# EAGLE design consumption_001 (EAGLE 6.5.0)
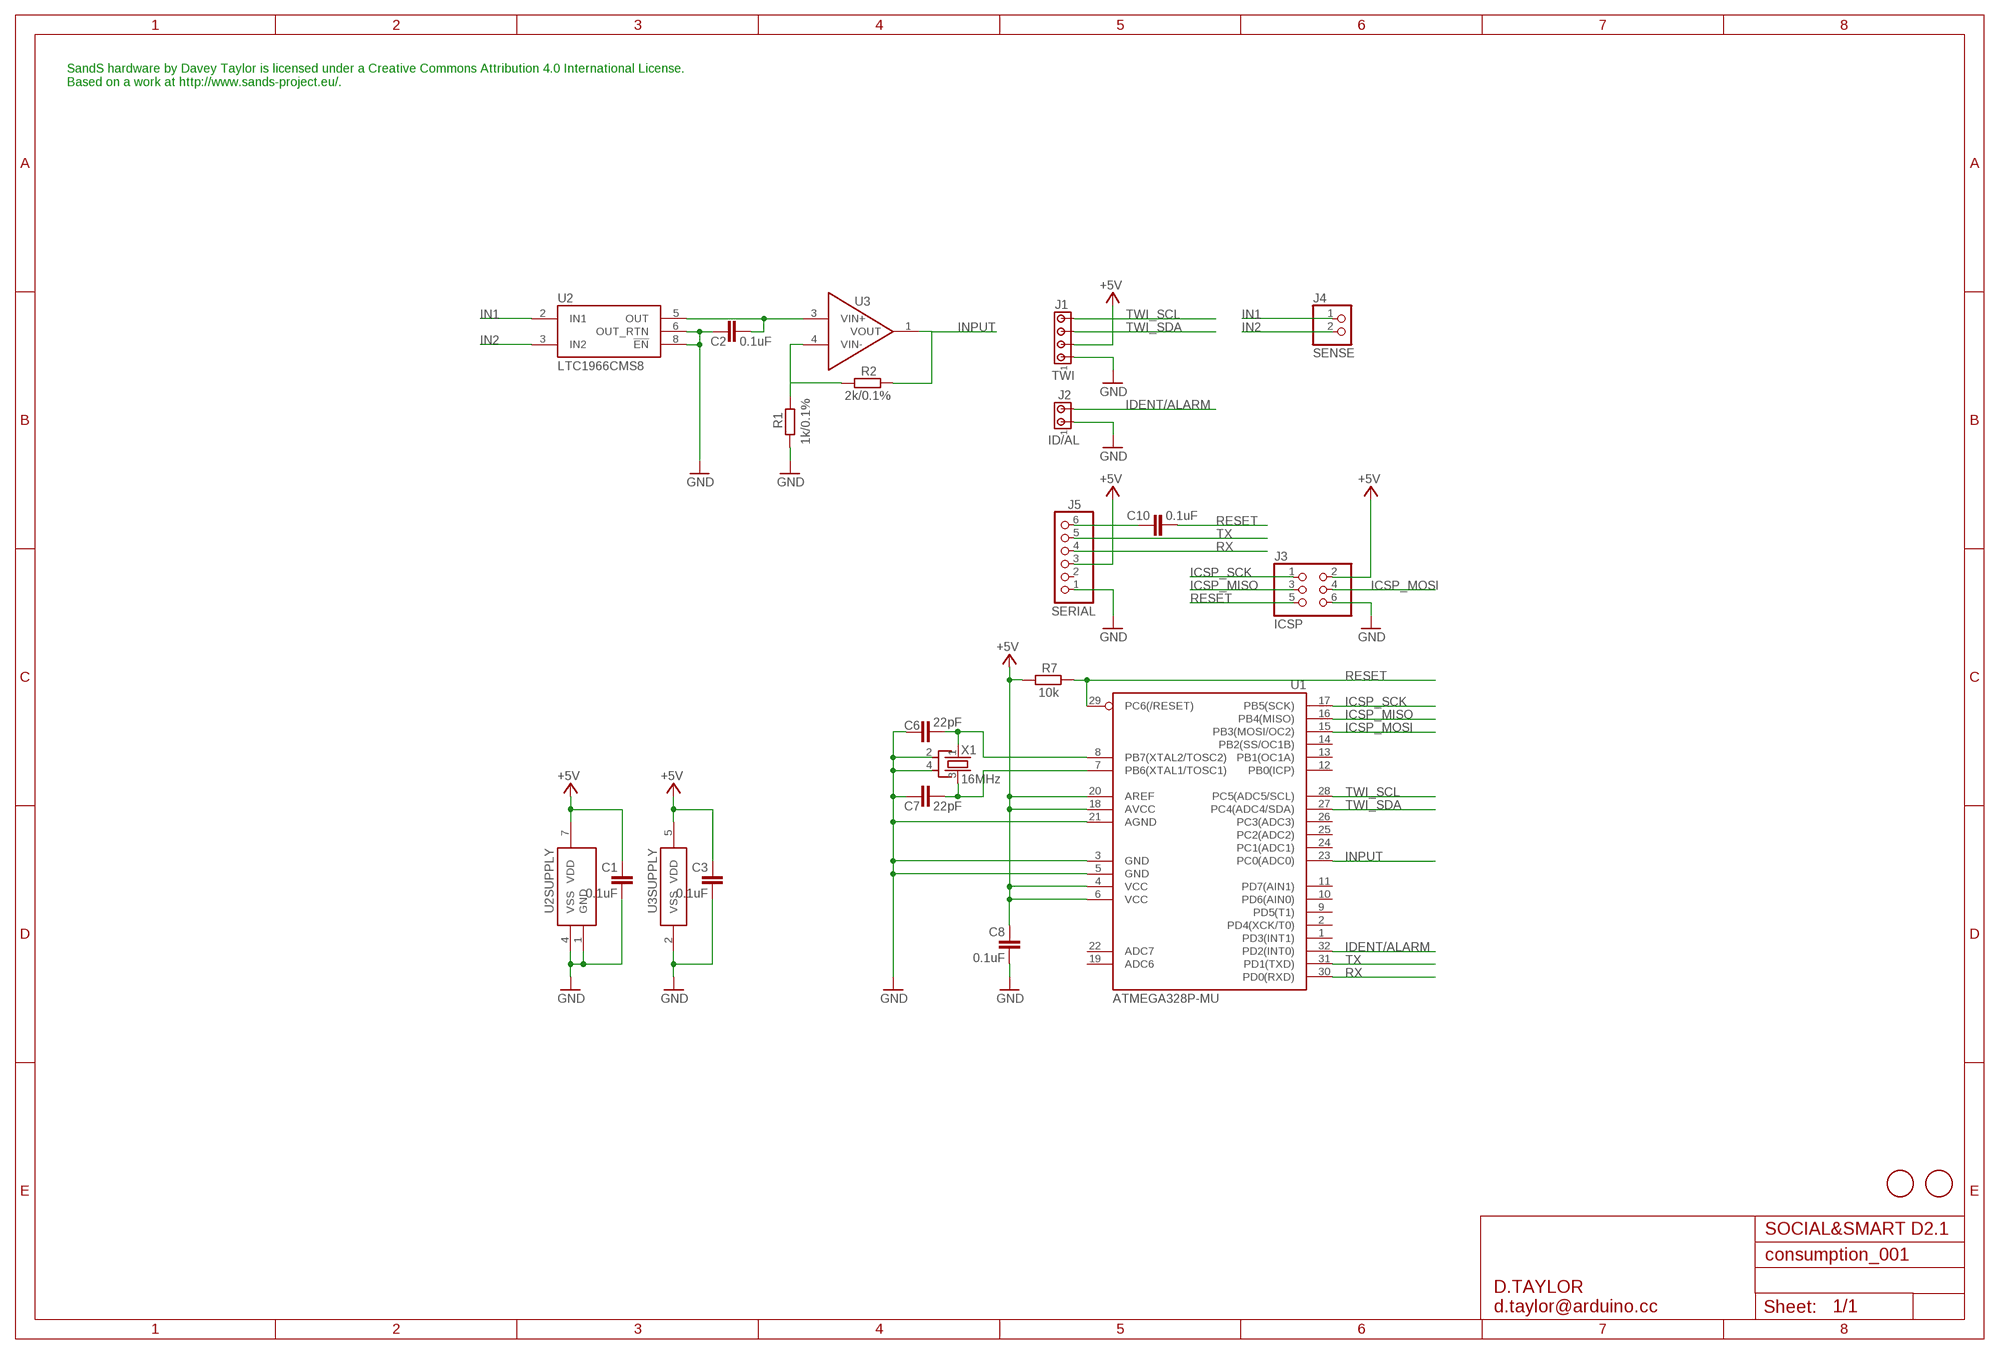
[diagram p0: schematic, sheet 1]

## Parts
C1  0.1uF  C-EUC0603  [C0603]
C2  0.1uF  C-EUC0603  [C0603]
C3  0.1uF  C-EUC0603  [C0603]
C6  22pF  C-EUC0603  [C0603]
C7  22pF  C-EUC0603  [C0603]
C8  0.1uF  C-EUC0603  [C0603]
C10  0.1uF  C-EUC0603  [C0603]
J1  TWI  MTA04-100  [10X04MTA]
J2  ID/AL  MTA02-100  [10X02MTA]
J3  ICSP  PINHD-2X3  [2X03]
J4  SENSE  MKDS_1,5/2-5,08  [MKDS1,5/2-5,08]
J5  SERIAL  PINHD-1X6  [1X06]
R1  1k/0.1%  R-EU_R0603  [R0603]
R2  2k/0.1%  R-EU_R0603  [R0603]
R7  10k  R-EU_R0603  [R0603]
U1  ATMEGA328P-MU  [MLF32-M1-A]
U2  LTC1966CMS8  [MSOP08]
U3  MCP6401-E/OT  [SOT-23-5]
U$5  FIDUCIALMOUNT  [FIDUCIA-MOUNT]
U$6  FIDUCIALMOUNT  [FIDUCIA-MOUNT]
X1  16MHz  CRYSTAL-KX7  [XTAL-3.2-2.5]

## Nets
+5V: C1.1 C3.1 C8.1 J1.2 J3.2 J5.3 R7.1 U1.4(VCC) U1.6(VCC) U1.18(AVCC) U1.20(AREF) U2.7(VDD) U3.5(VDD)
GND: C1.2 C2.1 C3.2 C6.1 C7.1 C8.2 J1.1 J2.1 J3.6 J5.1 R1.1 U1.3(GND) U1.5(GND) U1.21(AGND) U2.1(GND) U2.4(VSS) U2.6(OUT_RTN) U2.8(!EN!) U3.2(VSS) X1.2(SH1) X1.4(SH2)
ICSP_MISO: J3.3 U1.16(PB4(MISO))
ICSP_MOSI: J3.4 U1.15(PB3(MOSI/OC2))
ICSP_SCK: J3.1 U1.17(PB5(SCK))
IDENT/ALARM: J2.2 U1.32(PD2(INT0))
IN1: J4.1 U2.2(IN1)
IN2: J4.2 U2.3(IN2)
INPUT: R2.1 U1.23(PC0(ADC0)) U3.1(VOUT)
N$1: C2.2 U2.5(OUT) U3.3(VIN+)
N$2: R1.2 R2.2 U3.4(VIN-)
N$6: C6.2 U1.8(PB7(XTAL2/TOSC2)) X1.1(X1)
N$7: C7.2 U1.7(PB6(XTAL1/TOSC1)) X1.3(X2)
N$9: C10.1 J5.6
RESET: C10.2 J3.5 R7.2 U1.29(PC6(/RESET))
RX: J5.4 U1.30(PD0(RXD))
TWI_SCL: J1.4 U1.28(PC5(ADC5/SCL))
TWI_SDA: J1.3 U1.27(PC4(ADC4/SDA))
TX: J5.5 U1.31(PD1(TXD))
Unconnected: J5.2 U1.1(PD3(INT1)) U1.2(PD4(XCK/T0)) U1.9(PD5(T1)) U1.10(PD6(AIN0)) U1.11(PD7(AIN1)) U1.12(PB0(ICP)) U1.13(PB1(OC1A)) U1.14(PB2(SS/OC1B)) U1.19(ADC6) U1.22(ADC7) U1.24(PC1(ADC1)) U1.25(PC2(ADC2)) U1.26(PC3(ADC3))

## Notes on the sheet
- SandS hardware by Davey Taylor is licensed under a Creative Commons Attribution 4.0 International License.
  Based on a work at http://www.sands-project.eu/.
- SOCIAL&SMART D2.1
- D.TAYLOR
  d.taylor@arduino.cc

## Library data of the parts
C1-C3 C6-C8 C10 = rcl:C-EU: CAPACITOR, European symbol
J1 = con-amp:MTA04-100: AMP connector
J2 = con-amp:MTA02-100: AMP connector
J3 = pinhead:PINHD-2X3: PIN HEADER
J4 = d_taylor:MKDS_1,5/2-5,08: Screw terminal header
J5 = pinhead:PINHD-1X6: PIN HEADER
R1 R2 R7 = rcl:R-EU_: RESISTOR, European symbol
U1 = d_taylor:ATMEGA*: MICROCONTROLLER 8 Kbytes FLASH 1 kbytes SRAM 512 bytes EEPROM USART 6-channel 10 bit ADC 2-channel 8 bit ADC Source: avr.lbr
U2 = d_taylor:LTC1966*MS8: Precision Micropower Delta-Sigma RMS-to-DC Converter
U3 = d_taylor:MCP6401*
U$5 U$6 = SmartPrj:FIDUCIALMOUNT
X1 = d_taylor:CRYSTAL-KX7

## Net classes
1 PWR: width 0.406 mm, clearance 0.254 mm

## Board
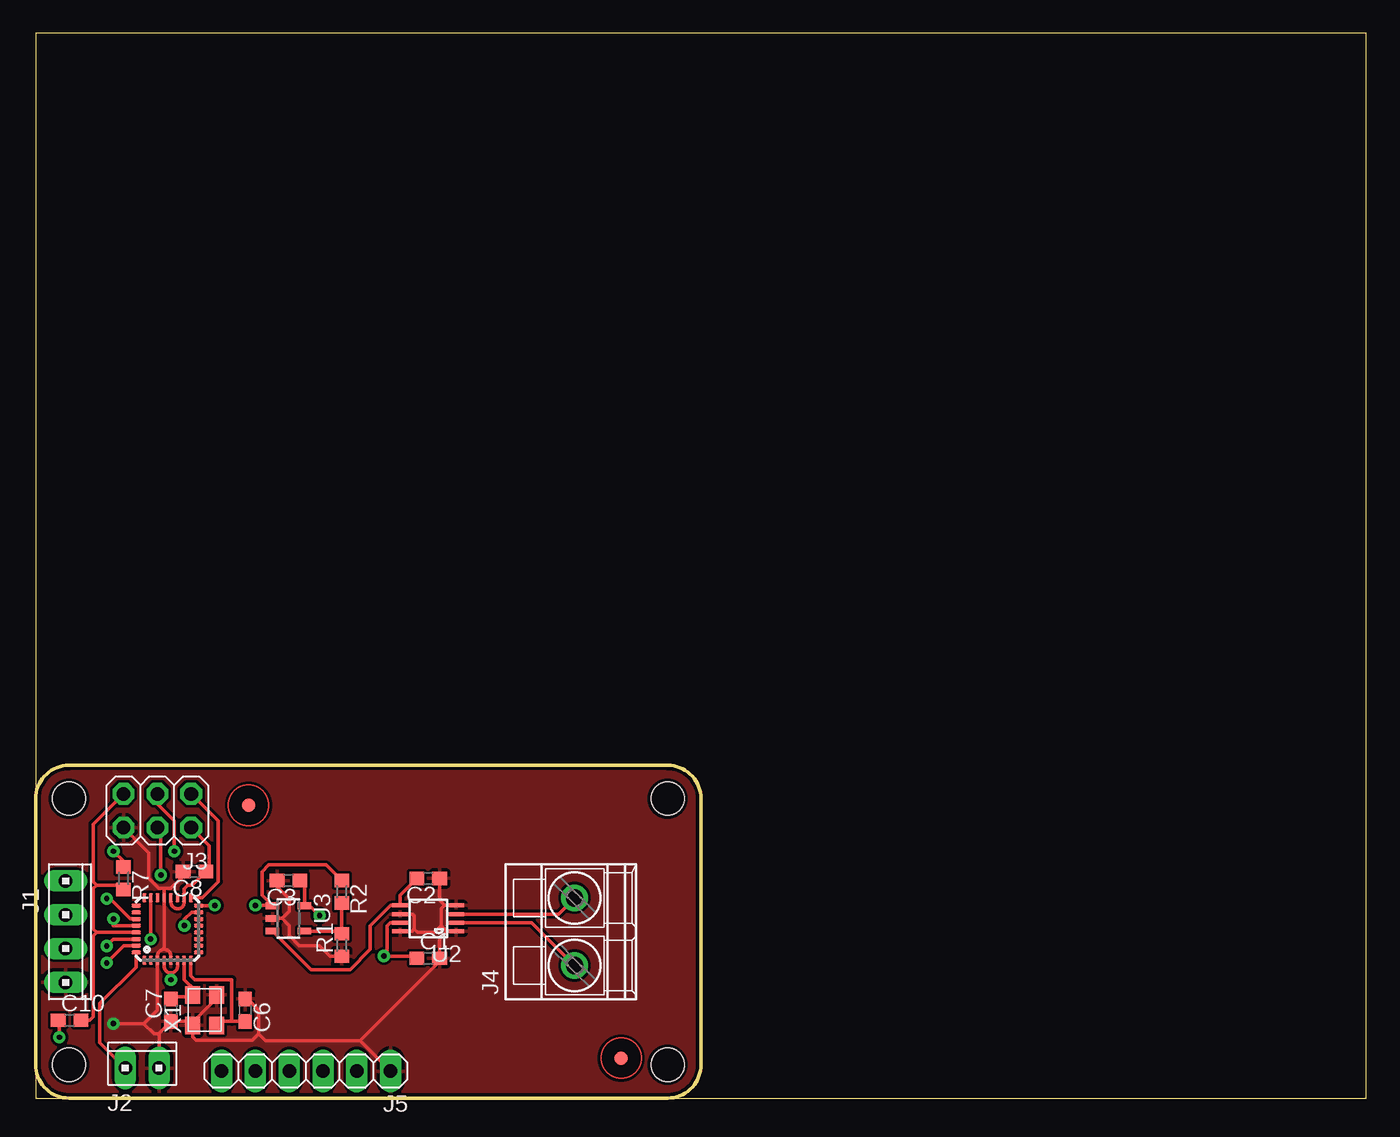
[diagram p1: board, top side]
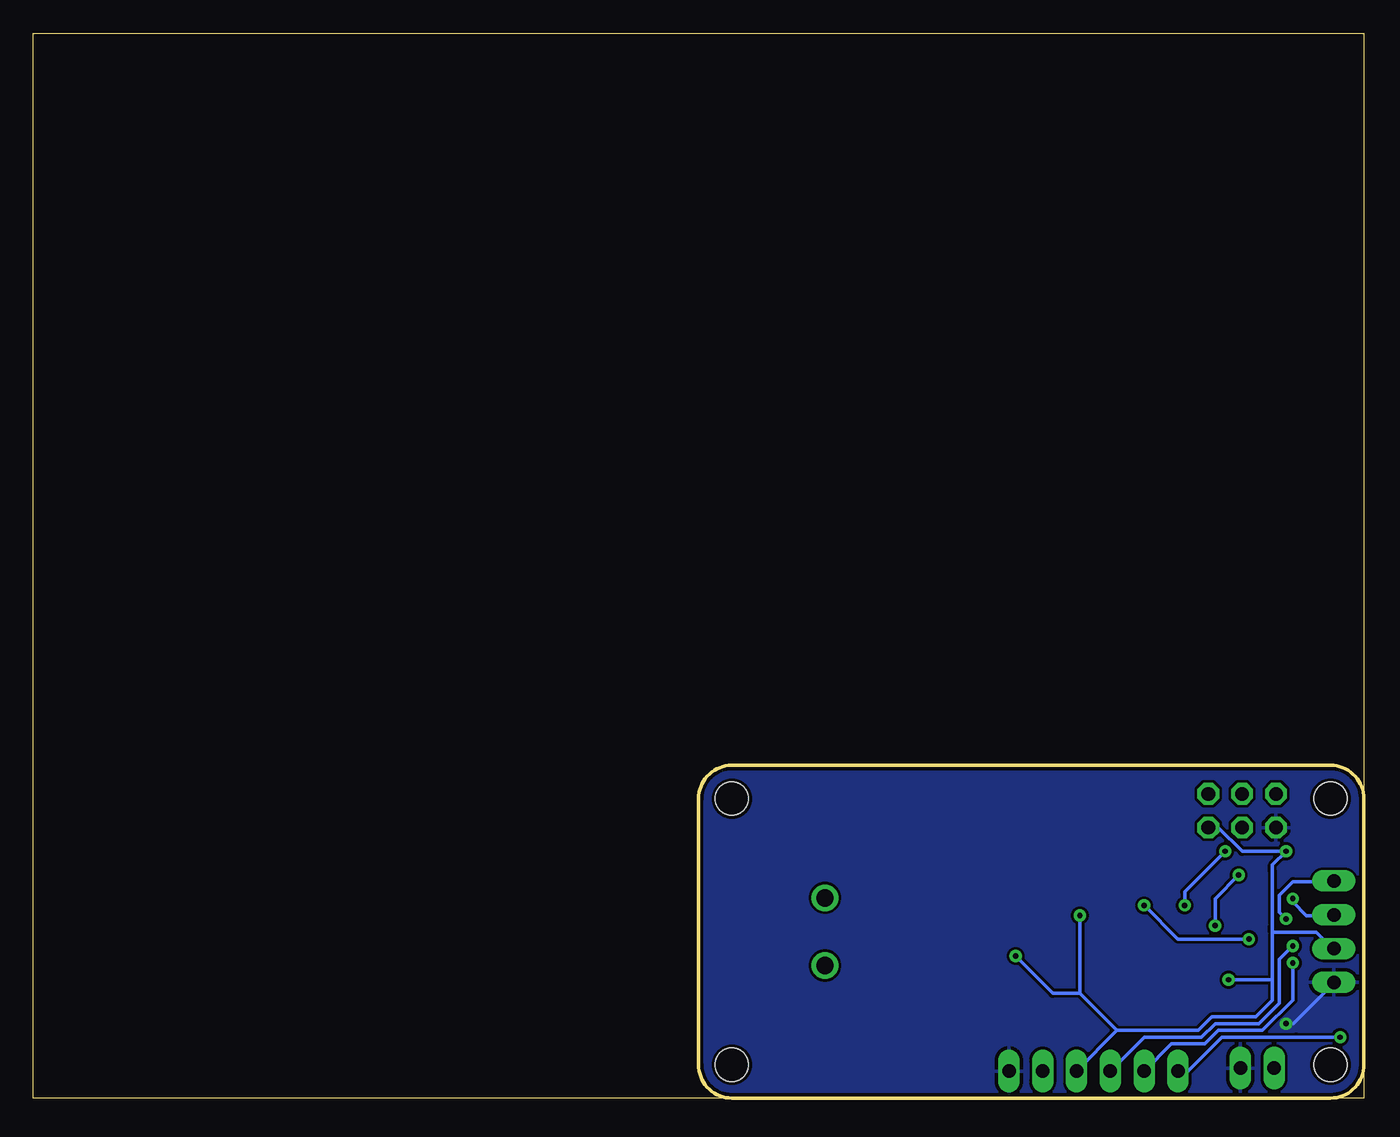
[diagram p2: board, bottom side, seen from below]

Size 100 x 80 mm. Coordinates in mm from the lower left corner, seen from the top.
Outline: 0,0 100,0 100,80 0,80 0,0
Outline: 2.5,0 47.5,0 arc90 50,2.5 50,22.5 arc90 47.5,25 2.5,25 arc90 0,22.5 0,2.5 arc90 2.5,0
Copper layers (1*16): Top 0.035mm / dielectric 1.5mm / Bottom 0.035mm
Design rules "smartprj-mini *": minimum track width 8mil, minimum drill 16mil, track to track 8mil, track to pad 8mil, pad to pad 0.200659375mm, via to via 8mil, smd to smd 4mil, copper to edge 10mil, drill to drill 8mil, minimum pad ring 12mil, minimum via ring 10mil, stop-mask expansion 2mil, vias tented up to drill 20mil, thermal gap 10mil
Holes 2.5 mm at 2.5,22.5 2.5,2.5 47.5,2.5 47.5,22.5

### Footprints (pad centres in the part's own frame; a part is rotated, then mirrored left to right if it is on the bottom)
C0603 = smd 1.1 x 1: 1 -0.85,0; 2 0.85,0
10X04MTA = drill 1.016 long: 1 3.81,0; 2 1.27,0; 3 -1.27,0; 4 -3.81,0
10X02MTA = drill 1.016 long: 1 1.27,0; 2 -1.27,0
2X03 = drill 1.016 octagon: 1 -2.54,-1.27; 2 -2.54,1.27; 3 0,-1.27; 4 0,1.27; 5 2.54,-1.27; 6 2.54,1.27
MKDS1,5/2-5,08 = drill 1.3 pad 2: 1 -2.54,0; 2 2.54,0
1X06 = drill 1.016 long: 1 -6.35,0; 2 -3.81,0; 3 -1.27,0; 4 1.27,0; 5 3.81,0; 6 6.35,0
R0603 = smd 1 x 1.1: 1 -0.85,0; 2 0.85,0
MLF32-M1-A = smd 0.7 x 0.3: 1 -2.35,1.75; 2 -2.35,1.25; 3 -2.35,0.75; 4 -2.35,0.25; 5 -2.35,-0.25; 6 -2.35,-0.75; 7 -2.35,-1.25; 8 -2.35,-1.75; 17 2.35,-1.75; 18 2.35,-1.25; 19 2.35,-0.75; 20 2.35,-0.25; 21 2.35,0.25; 22 2.35,0.75; 23 2.35,1.25; 24 2.35,1.75 | smd 0.3 x 0.7: 9 -1.75,-2.35; 10 -1.25,-2.35; 11 -0.75,-2.35; 12 -0.25,-2.35; 13 0.25,-2.35; 14 0.75,-2.35; 15 1.25,-2.35; 16 1.75,-2.35; 25 1.75,2.35; 26 1.25,2.35; 27 0.75,2.35; 28 0.25,2.35; 29 -0.25,2.35; 30 -0.75,2.35; 31 -1.25,2.35; 32 -1.75,2.35
MSOP08 = smd 0.3 x 1.2: 1 -0.976,-2.113; 2 -0.326,-2.113; 3 0.324,-2.113; 4 0.974,-2.113; 5 0.974,2.112; 6 0.324,2.112; 7 -0.326,2.112; 8 -0.976,2.112
SOT-23-5 = smd 0.5 x 1: 1 -0.95,-1.2; 2 0,-1.2; 3 0.95,-1.2; 4 0.95,1.2; 5 -0.95,1.2
FIDUCIA-MOUNT = smd 1.016 x 1.016: P$1 0,0
XTAL-3.2-2.5 = smd 1.3 x 1.1: 1 -1.15,-0.9; 2 1.15,-0.9; 3 1.15,0.9; 4 -1.15,0.9

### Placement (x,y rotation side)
C1  29.5,10.5 0 top
C2  29.5,16.5 180 top
C3  19,16.34 180 top
C6  15.75,6.6 270 top
C7  10.16,6.6 90 top
C8  11.94,17.02 180 top
C10  2.54,5.84 0 top
J1  2.25,12.5 270 top
J2  8,2.25 0 top
J3  9.14,21.59 180 top
J4  40.5,12.5 90 top
J5  20.32,2.03 180 top
R1  23,11.5 90 top
R2  23,15.5 270 top
R7  6.6,16.51 270 top
U1  9.91,12.7 90 top
U2  29.5,13.5 90 top
U3  19,13.5 270 top
U$5  16,22 0 top
U$6  44,3 0 top
X1  12.7,6.6 90 top

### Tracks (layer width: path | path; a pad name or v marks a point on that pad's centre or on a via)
+5V  (via drill 0.41)
  Top 0.254: 11.18,15.32 U1.18 | 11.18,15.05 U1.18 | R7.1 6.6,17.78 v5.84,18.54 | U1.4 9.66,9.9 arc90 10.16,9.4 | 10.16,9.4 arc90 10.66,9.89 U1.6 | 10.16,9.4 v10.16,8.89 | U1.18 11.16,15.64 11.16,15.73 11.43,16 11.77,16 C8.1 13.04,17.27 13.04,18.96 J3.2 | U1.18 11.16,14.71 arc-90 10.67,14.22 arc-90 10.16,14.74 U1.20 | C3.1 20.2,15.99 U3.5 20.6,14.45 v21.34,13.72 | U2.7 26.64,13.17 26.42,12.95 26.42,12.19 26.42,10.92 v26.16,10.67 28.48,10.67 C1.1
  Bottom 0.254: 18.54,5.08 12.45,5.08 11.43,6.1 8.13,6.1 7.37,6.86 6.86,7.37 6.86,8.89 | 6.86,15.75 6.86,15.49 | 6.86,15.49 6.86,12.95 | 6.86,12.95 6.86,12.45 | 6.86,12.45 3.56,12.45 2.25,11.18 J1.2 | 6.86,12.45 6.86,12.95 | 6.86,12.95 6.86,8.89 | 6.86,15.75 6.86,17.02 6.86,17.53 v5.84,18.54 9.14,18.54 10.92,20.32 J3.2 | J5.3 18.54,5.08 | v10.16,8.89 6.86,8.89 | 6.86,15.75 6.86,15.49 | v21.34,13.72 21.34,7.87 | 21.34,7.87 18.54,5.08 | 21.34,7.87 23.37,7.87 v26.16,10.67
GND  (via drill 0.41)
  Top 0.254: 13.85,7.62 X1.2 13.6,7.5 12.7,6.6 11.8,5.7 X1.4 | 12.05,5.75 X1.4 | 10.16,10.16 U1.5 10.16,10.68 arc90 9.66,11.18 | 9.14,10.35 U1.3 9.14,10.35 | 9.66,11.18 9.65,11.18 U1.21 9.65,15.75 | 9.14,10.35 9.14,6.6 8.13,5.59 | J2.1 9.27,4.06 9.27,4.35 9.27,4.83 | X1.4 11.8,5.75 C7.1 9.27,4.86 9.27,4.83 | 9.14,10.35 9.14,10.66 arc-90 9.66,11.18 | C6.1 15.91,7.45 16.76,6.6 16.76,4.83 | 16.76,4.83 16.26,4.35 12.05,4.35 11.8,4.6 X1.4 | J3.6 8.5,18.42 8.5,16.5 9.25,15.75 9.65,15.75 | 9.65,15.75 10.16,15.75 10.92,16.51 10.92,16.85 C8.2 | 8.13,5.59 v5.84,5.59 | 8.13,5.59 8.89,4.83 9.27,4.83 | U2.4 30.73,14.48 | 30.73,14.48 30.48,14.22 30.48,12.95 | U2.1 30.91,12.52 | 30.91,12.52 30.48,12.95 | 30.91,12.52 30.35,11.96 C1.2 30.35,10.28 24.38,4.32 | 30.73,14.48 30.35,14.86 C2.1 | U2.6 28.34,13.82 28.45,13.72 28.45,12.7 | U2.8 28.27,12.52 28.45,12.7 | 28.45,12.7 28.7,12.45 29.97,12.45 30.48,12.95 | 16.76,4.83 17.27,4.32 24.38,4.32 | 24.38,4.32 J5.1 | R1.1 22.12,10.65 21.34,11.43 19.84,11.43 19.81,11.46 19.08,12.19 19.05,12.19 19.05,12.95 18.5,13.5 | U3.2 18.5,13.5 | C3.2 18.15,15.89 19.05,14.99 19.05,14.05 18.5,13.5
  Bottom 0.254: 2.25,8.64 5.3,5.59 v5.84,5.59
  pour Top: 0.5,22.5 arc-90 2.5,24.5 47.5,24.5 arc-90 49.5,22.5 49.5,2.5 arc-90 47.5,0.5 2.5,0.5 arc-90 0.5,2.5
  pour Bottom: 0.5,22.5 arc-90 2.5,24.5 47.5,24.5 arc-90 49.5,22.5 49.5,2.5 arc-90 47.5,0.5 2.5,0.5 arc-90 0.5,2.5
ICSP_MISO  (via drill 0.41)
  Top 0.254: J3.3 9.14,22.1 10.41,20.83 10.41,19.56 v10.41,18.54 | v13.46,14.48 13.72,14.45 U1.16
  Bottom 0.254: v10.41,18.54 13.46,15.49 v13.46,14.48
ICSP_MOSI  (via drill 0.41)
  Top 0.254: J3.4 9.4,20.07 v9.4,16.76 | U1.15 11.7,13.95 11.18,13.42 v11.18,12.95
  Bottom 0.254: v9.4,16.76 11.18,14.99 v11.18,12.95
ICSP_SCK
  Top 0.254: U1.17 12.51,15.05 13.72,16.26 13.72,20.83 J3.1
IDENT/ALARM
  Top 0.254: J2.2 4.83,4.16 4.83,7.11 7.56,9.84 U1.32
IN1
  Top 0.254: J4.1 37.29,13.17 U2.2
IN2
  Top 0.254: J4.2 39.28,13.82 U2.3
INPUT  (via drill 0.41)
  Top 0.254: U1.23 8.66,11.96 v8.64,11.94 | R2.1 21.82,17.53 17.53,17.53 17.02,17.02 17.02,15.24 U3.1 17.77,14.48 v16.51,14.48
  Bottom 0.254: v8.64,11.94 13.97,11.94 v16.51,14.48
N$1
  Top 0.254: C2.2 27.39,15.24 U2.5 26.67,14.48 25.15,12.95 25.15,11.18 23.62,9.65 20.83,9.65 20.7,9.65 U3.3
N$2
  Top 0.254: U3.4 22.8,12.55 R1.2 R2.2
N$6
  Top 0.254: C6.2 14.73,5.75 | 14.73,5.75 14.73,8.89 11.94,8.89 11.68,9.14 11.66,9.17 U1.8 | 14.73,5.75 13.9,5.75 X1.1
N$7
  Top 0.254: C7.2 10.16,7.62 12.05,7.62 X1.3 11.94,7.75 11.94,8.13 11.16,8.89 U1.7
N$9  (via drill 0.41)
  Top 0.254: v1.78,4.57 1.78,5.84 C10.1
  Bottom 0.254: J5.6 13.21,2.03 10.67,4.57 5.08,4.57 v1.78,4.57
RESET
  Top 0.254: U1.29 5.84,12.45 4.57,12.45 | 4.57,12.45 4.32,12.7 4.32,15.75 4.57,16 | C10.2 4.06,5.84 4.32,6.1 4.32,12.19 4.57,12.45 | R7.2 6.6,16 4.57,16 | 4.57,16 4.32,16.26 4.32,19.56 4.32,20.57 J3.5
RX  (via drill 0.41)
  Top 0.254: U1.30 7.56,11.94 5.84,11.94 v5.33,11.43
  Bottom 0.254: v5.33,11.43 6.35,10.41 6.35,7.11 6.86,6.6 7.87,5.59 11.18,5.59 12.19,4.57 16.51,4.57 J5.4
TWI_SCL  (via drill 0.41)
  Top 0.254: U1.28 5.84,12.95 v5.84,13.46
  Bottom 0.254: v5.84,13.46 6.35,13.97 6.35,15.24 5.33,16.26 2.29,16.26 2.29,16.31 J1.4
TWI_SDA  (via drill 0.41)
  Top 0.254: v5.33,14.99 5.59,14.99 7.11,13.46 7.56,13.46 U1.27
  Bottom 0.254: J1.3 2.25,13.72 4.32,13.72 5.33,14.73 v5.33,14.99
TX  (via drill 0.41)
  Top 0.254: U1.31 6.6,11.45 v5.33,10.16
  Bottom 0.254: v5.33,10.16 5.33,7.37 7.62,5.08 10.92,5.08 11.94,4.06 14.48,4.06 J5.5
